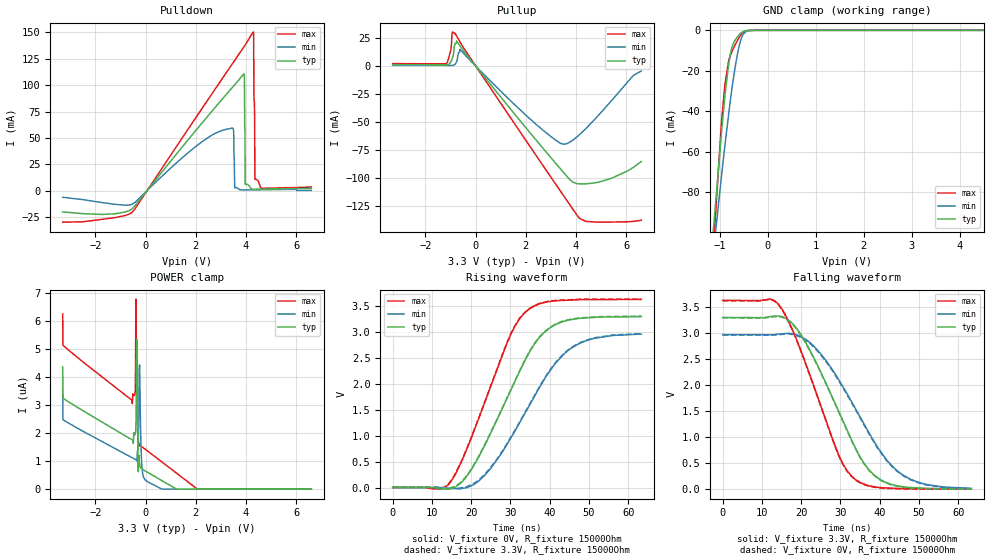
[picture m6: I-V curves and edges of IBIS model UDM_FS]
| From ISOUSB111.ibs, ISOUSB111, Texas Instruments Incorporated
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[Model]   UDM_FS
Model_type   I/O
Polarity   Non-Inverting
Enable   Active-Low
Vinl = 0.8
Vinh = 2
Vmeas = 1.65
Vref = 1.65
Cref = 7pF
Rref = 15000
|   typ   min   max
C_comp   8pF   5pF   10pF
[Voltage Range]   3.3   2.97   3.63
[Temperature Range]   27   150   -40
[Pullup Reference]   3.3   2.97   3.63
[Pulldown Reference]   -0   -0   -0
[Power Clamp Reference]   3.3   2.97   3.63
[GND Clamp Reference]   0   0   0
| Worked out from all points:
|   slope of the pulldown table from 0 to 0.495 V, typ, clamps not added: 33.7 ohm
|   slope of the pullup table from 0 to 0.495 V, typ, clamps not added: 35.8 ohm
|   GND clamp passes 1 mA (typ) near -0.54 V on its own axis
|   falling waveform, V_fixture 3.3V, R_fixture 15000Ohm: 20-80 % time 12.3ns typ, 14.2ns min, 10.5ns max; typ from 3.3 V to 0.008 V
|   rising waveform, V_fixture 0V, R_fixture 15000Ohm: 20-80 % time 12.6ns typ, 14.1ns min, 11ns max; typ from 0 V to 3.29 V
|   rising waveform, V_fixture 3.3V, R_fixture 15000Ohm: 20-80 % time 12.7ns typ, 14.1ns min, 11ns max; typ from 0.007 V to 3.3 V
|   falling waveform, V_fixture 0V, R_fixture 15000Ohm: 20-80 % time 12.3ns typ, 14.2ns min, 10.5ns max; typ from 3.29 V to 0 V
[Pulldown]
|   Voltage   I(typ)   I(min)   I(max)
-3.3V     -19.93mA   -6.107mA   -29.66mA
-537.9mV  -16.94mA   -12.7mA    -20.3mA
3.452V    97.68mA    59.35mA    120.1mA
3.551V    100.4mA    2.79mA     123.5mA
3.917V    110.6mA    791.1uA    136.2mA
3.937V    107.5mA    798uA      136.9mA
3.967V    6.141mA    808.4uA    138mA
4.283V    1.56mA     916.9uA    150.2mA
4.303V    1.492mA    923.6uA    149.6mA
4.343V    1.509mA    936.8uA    69.22mA
4.353V    1.513mA    940.1uA    10.96mA
6.6V      2.508mA    452.9uA    3.524mA
[GND Clamp]
|   Voltage   I(typ)   I(min)   I(max)
-3.3V     -1.286A    -1.12A     -1.579A
-1.3V     -145.3mA   -147.2mA   -170.6mA
-973.5mV  -52.59mA   -73.66mA   -47.69mA
-894.3mV  -32.06mA   -56.82mA   -26.49mA
-815.1mV  -16.5mA    -41.06mA   -14.88mA
-785.4mV  -12.23mA   -35.46mA   -12.65mA
-735.9mV  -7.575mA   -26.62mA   -9.854mA
-627mV    -3.033mA   -10.97mA   -4.745mA
-567.6mV  -1.539mA   -5.066mA   -2.489mA
-498.3mV  -471.8uA   -1.572mA   -746.7uA
-260.7mV  0A         -5.306uA   0A
6.6V      0A         0A         0A
[Pullup]
|   Voltage   I(typ)   I(min)   I(max)
-3.3V     1.142mA    462.6uA    2.095mA
-1.181V   1.061mA    442uA      1.922mA
-993.3mV  3.358mA    441.5uA    13.7mA
-933.9mV  6.314mA    531.1uA    29.51mA
-815.1mV  20.17mA    1.584mA    29.25mA
-627mV    18.16mA    15.03mA    21.83mA
1.957V    -54.04mA   -43.08mA   -65.14mA
3.501V    -95.32mA   -70.05mA   -116.1mA
3.868V    -103.9mA   -66.47mA   -128mA
4.392V    -105.6mA   -56.06mA   -139.2mA
5.412V    -100.6mA   -31.15mA   -139.8mA
6.6V      -85.55mA   -4.486mA   -138.2mA
[POWER Clamp]
|   Voltage   I(typ)   I(min)   I(max)
-3.3V     4.356uA    3.599uA    6.245uA
-3.29V    3.24uA     2.477uA    5.129uA
-528mV    1.759uA    1.119uA    3.053uA
-409.2mV  1.977uA    1.064uA    3.528uA
-379.5mV  2.534uA    1.044uA    6.78uA
-349.8mV  5.335uA    1.011uA    3.323uA
-290.4mV  625.9nA    1.782uA    1.767uA
-250.8mV  987.2nA    4.223uA    1.563uA
-171.6mV  742.1nA    1.25uA     1.531uA
-82.5mV   684.7nA    428.7nA    1.471uA
2.056V    0A         0A         4.456nA
6.6V      0A         0A         0A
[Ramp]
R_load = 15000
|   typ   min   max
dV/dt_r   1.97313/1.26192e-08   1.77083/1.40324e-08   2.1712/1.09691e-08
dV/dt_f   1.97353/1.22096e-08   1.77092/1.41056e-08   2.17144/1.04715e-08
[Falling Waveform]
V_fixture = 3.3V
V_fixture_min = 2.97V
V_fixture_max = 3.63V
R_fixture = 15000Ohm
C_fixture = 0F
|   Time   V(typ)   V(min)   V(max)
0s        3.297V     2.968V     3.626V
12.09ns   3.313V     2.966V     3.651V
14.66ns   3.322V     2.98V      3.508V
18.36ns   3.132V     2.974V     2.956V
23.41ns   2.494V     2.732V     1.94V
29.8ns    1.452V     2.071V     611.3mV
33.82ns   791.7mV    1.546V     184.7mV
38.3ns    290.3mV    950.3mV    49.6mV
46.09ns   44.79mV    264.6mV    10.76mV
63.33ns   7.77mV     16.09mV    6.866mV
[Rising Waveform]
V_fixture = 0V
V_fixture_min = 0V
V_fixture_max = 0V
R_fixture = 15000Ohm
C_fixture = 0F
|   Time   V(typ)   V(min)   V(max)
0s        7.357nV    283.2nV    6.487nV
12.09ns   -26.05mV   -1.027mV   -31.65mV
14.66ns   -27.01mV   -14.92mV   98.06mV
18.36ns   166.2mV    -9.284mV   647.7mV
23.41ns   806mV      231.7mV    1.63V
30.23ns   1.895V     971.2mV    2.971V
34.59ns   2.572V     1.549V     3.424V
40.03ns   3.071V     2.241V     3.579V
45.63ns   3.232V     2.687V     3.608V
63.33ns   3.289V     2.951V     3.619V
[Rising Waveform]
V_fixture = 3.3V
V_fixture_min = 2.97V
V_fixture_max = 3.63V
R_fixture = 15000Ohm
C_fixture = 0F
|   Time   V(typ)   V(min)   V(max)
0s        7.485mV    8.596mV    6.856mV
12.09ns   -13.82mV   7.096mV    -17.8mV
14.66ns   -7.906mV   -9.264mV   111.8mV
18.36ns   181.9mV    8.119mV    659.8mV
23.41ns   819.4mV    250.8mV    1.641V
30.23ns   1.907V     987.8mV    2.981V
34.59ns   2.584V     1.566V     3.432V
40.03ns   3.081V     2.259V     3.587V
45.63ns   3.241V     2.699V     3.615V
63.33ns   3.296V     2.96V      3.626V
[Falling Waveform]
|Gnd
V_fixture = 0V
V_fixture_min = 0V
V_fixture_max = 0V
R_fixture = 15000Ohm
C_fixture = 0F
|   Time   V(typ)   V(min)   V(max)
0s        3.289V     2.959V     3.619V
12.09ns   3.304V     2.957V     3.64V
14.66ns   3.309V     2.969V     3.497V
18.36ns   3.117V     2.962V     2.945V
23.41ns   2.481V     2.713V     1.929V
29.73ns   1.451V     2.058V     613.7mV
33.77ns   788mV      1.534V     179.6mV
38.3ns    279.9mV    931.6mV    40.96mV
46.09ns   36.64mV    251.2mV    3.861mV
63.33ns   271.3uV    7.115mV    10.05uV
